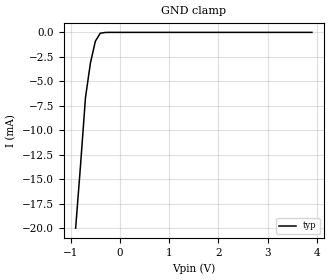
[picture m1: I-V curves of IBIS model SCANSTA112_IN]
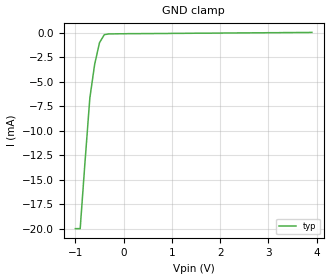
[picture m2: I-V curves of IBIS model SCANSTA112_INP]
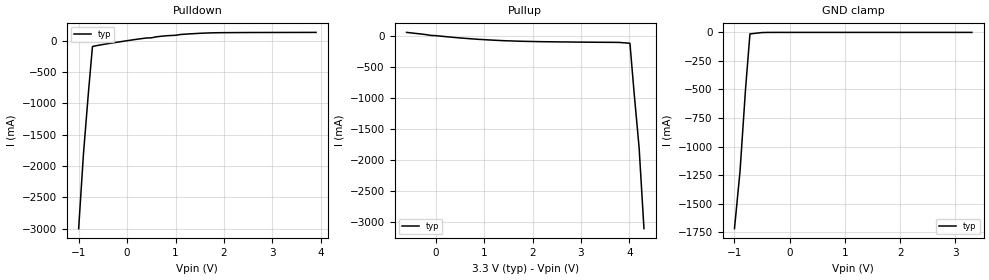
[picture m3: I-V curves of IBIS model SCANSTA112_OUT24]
| Texas Instruments Incorporated
| SCANSTA112 7-Port Multidrop IEEE 1149.1 (JTAG) Multiplexer
| Marketing part#   Voltage Range   Package-type   #pins/pkg drawing
| SCANSTA112VS   3.0V - 3.6V   TQFP   100/NEZ
| SCANSTA112SM   3.0V - 3.6V   NFBGA   100/NZD
[IBIS Ver]   4.1
[File name]   scansta112.ibs
[File Rev]   1.0
[Date]   04/11/13
[Source]   File originated at National Semiconductor Corporation
   System Test Access Group/Enhanced Solutions Division
   All data based on simulations, except where specified.
[Notes]   Revision History
   Rev 1.0: 04/11/2013
   - Model based on SCANSTA101 buffer models. Only nom available.
   Since these models are based on a related device, accuracy is not assured.
[Disclaimer]  This model is designed as an aid for customers of Texas Instruments
 TI and its licensors and suppliers make no warranties, either expressed
 or implied, with respect to this  model, including the warranties of
 merchantability or fitness for a particular purpose.
 The model is provided solely on an "as is" basis. The entire risk as to
 its quality and performance is with the customer.
[Copyright] (C)Copyright 2013 Texas Instruments Incorporated.
   All rights reserved.
| Component SCANSTA112NZD 100 pin NFBGA
[Component]  SCANSTA112NZD
[Manufacturer]  Texas Instruments
[Package]
|   typ   min   max
R_pkg   65.0m   NA   NA
L_pkg   1.50nH   NA   NA
C_pkg   0.08pF   NA   NA
[Pin]   signal_name   model_name   R_pin   L_pin   C_pin
A1   S0   SCANSTA112_IN
A2   TCK06   SCANSTA112_OUT24
A3   TDO06   SCANSTA112_OUT12
A4   VCC   POWER
A5   TMS04   SCANSTA112_OUT24
A6   GND   GND
A7   TCK04   SCANSTA112_OUT24
A8   TMS04   SCANSTA112_OUT24
A9   VCC   POWER
A10   TDO03   SCANSTA112_OUT12
B1   GND   GND
B2   S1   SCANSTA112_IN
B3   GND   GND
B4   TDI06   SCANSTA112_INP
B5   TCK04   SCANSTA112_OUT24
B6   TDO05   SCANSTA112_OUT12
B7   TRST04B   SCANSTA112_OUT24
B8   TCK03   SCANSTA112_OUT24
B9   TMS03   SCANSTA112_OUT24
B10   TRIST02   SCANSTA112_OUT12
C1   S7   SCANSTA112_IN
C2   S3   SCANSTA112_IN
C3   VCC   POWER
C4   TMS06   SCANSTA112_OUT24
C5   TRST05B   SCANSTA112_OUT24
C6   TDO04   SCANSTA112_OUT12
C7   TDI04   SCANSTA112_INP
C8   GND   GND
C9   VCC   POWER
C10   TCK02   SCANSTA112_OUT24
D1   ADDMASK   SCANSTA112_IN
D2   TRANS   SCANSTA112_IN
D3   S5   SCANSTA112_IN
D4   S4   SCANSTA112_IN
D5   TRST06B   SCANSTA112_OUT24
D6   TRST03B   SCANSTA112_OUT24
D7   TRIST03   SCANSTA112_OUT12
D8   TRST02B   SCANSTA112_OUT24
D9   TMS02   SCANSTA112_OUT24
D10   GND   GND
E1   VCC   POWER
E2   LSPsel0   SCANSTA112_IN
E3   S6   SCANSTA112_IN
E4   S2   SCANSTA112_IN
E5   LSPsel1   SCANSTA112_IN
E6   TDI05   SCANSTA112_INP
E7   TDI03   SCANSTA112_INP
E8   TDO02   SCANSTA112_OUT12
E9   TDI02   SCANSTA112_INP
E10   A101   SCANSTA112_IN
F1   OE_B   SCANSTA112_IN
F2   LSPsel2   SCANSTA112_IN
F3   LSPsel3   SCANSTA112_IN
F4   SB/SB   SCANSTA112_IN
F5   A0B1   SCANSTA112_INP
F6   A001   SCANSTA112_IN
F7   RESETB   SCANSTA112_IN
F8   TCK01   SCANSTA112_OUT24
F9   Y001   SCANSTA112_OUT12
F10   VCC   POWER
G1   GND   GND
G2   LSPsel4   SCANSTA112_IN
G3   LSPsel6   SCANSTA112_IN
G4   TRSTB0B   SCANSTA112_IO24
G5   A0B0   SCANSTA112_INP
G6   A1B1   SCANSTA112_INP
G7   TDO01   SCANSTA112_OUT12
G8   TMS01   SCANSTA112_OUT24
G9   Y101   SCANSTA112_OUT12
G10   TRIST01   SCANSTA112_OUT12
H1   LSPsel5   SCANSTA112_IN
H2   VCC   POWER
H3   GND   GND
H4   TMSB0   SCANSTA112_IO24
H5   A1B0   SCANSTA112_INP
H6   TRSTB1B   SCANSTA112_IO24
H7   TRISTB1   SCANSTA112_OUT12
H8   VCC   POWER
H9   TDI01   SCANSTA112_INP
H10   TRST01B   SCANSTA112_OUT24
J1   MPseLB1   SCANSTA112_IN
J2   TDOB0   SCANSTA112_IO12
J3   TCKB0   SCANSTA112_IO24
J4   Y1B0   SCANSTA112_OUT12
J5   TDOB1   SCANSTA112_IO12
J6   TCKB1   SCANSTA112_IO24
J7   TMSB1   SCANSTA112_IO24
J8   GND   GND
J9   TLR_TRST6   SCANSTA112_IN
J10   GND   GND
K1   TDIB0   SCANSTA112_INP
K2   VCC   POWER
K3   TRISTB0   SCANSTA112_OUT12
K4   Y0B0   SCANSTA112_OUT12
K5   GND   GND
K6   TDIB1   SCANSTA112_INP
K7   VCC   POWER
K8   Y1B1   SCANSTA112_OUT12
K9   Y0B1   SCANSTA112_OUT12
K10   TLR_TRST   SCANSTA112_IN
| Component SCANSTA112NEZ 100 pin TQFP
[Component]  SCANSTA112NEZ
[Manufacturer]  Texas Instruments
[Package]
|   typ   min   max
R_pkg   65.0m   NA   NA
L_pkg   1.50nH   NA   NA
C_pkg   0.08pF   NA   NA
[Pin]   signal_name   model_name   R_pin   L_pin   C_pin
1   S0   SCANSTA112_IN
2   S1   SCANSTA112_IN
3   VDD   POWER
4   S2   SCANSTA112_IN
5   S3   SCANSTA112_IN
6   S4   SCANSTA112_IN
7   S5   SCANSTA112_IN
8   GND   GND
9   S6   SCANSTA112_IN
10   S7   SCANSTA112_IN
11   ADDMASK   SCANSTA112_IN
12   TRANS   SCANSTA112_IN
13   VDD   POWER
14   OE_B   SCANSTA112_IN
15   LSPsel0   SCANSTA112_IN
16   LSPsel1   SCANSTA112_IN
17   LSPsel2   SCANSTA112_IN
18   GND   GND
19   LSPsel3   SCANSTA112_IN
20   LSPsel4   SCANSTA112_IN
21   LSPsel5   SCANSTA112_IN
22   LSPsel6   SCANSTA112_IN
23   VDD   POWER
24   MPseLB1   SCANSTA112_IN
25   SB/SB   SCANSTA112_IN
26   TDIB0   SCANSTA112_INP
27   TDOB0   SCANSTA112_IO12
28   GND   GND
29   A0B0   SCANSTA112_INP
30   TCKB0   SCANSTA112_IO24
31   TRSTB0B   SCANSTA112_IO24
32   TMSB0   SCANSTA112_IO24
33   VDD   POWER
34   A1B0   SCANSTA112_INP
35   TRISTB0   SCANSTA112_OUT12
36   Y0B0   SCANSTA112_OUT12
37   Y1B0   SCANSTA112_OUT12
38   GND   GND
39   TDIB1   SCANSTA112_INP
40   TDOB1   SCANSTA112_IO12
41   A0B1   SCANSTA112_INP
42   TCKB1   SCANSTA112_IO24
43   VCC   POWER
44   TRSTB1B   SCANSTA112_IO24
45   TMSB1   SCANSTA112_IO24
46   Y1B1   SCANSTA112_OUT12
47   TRISTB1   SCANSTA112_OUT12
48   GND   GND
49   Y0B1   SCANSTA112_OUT12
50   A1B1   SCANSTA112_INP
51   TLR_TRST   SCANSTA112_IN
52   TLR_TRST6   SCANSTA112_IN
53   VCC   POWER
54   RESETB   SCANSTA112_IN
55   TDI01   SCANSTA112_INP
56   TDO01   SCANSTA112_OUT12
57   TMS01   SCANSTA112_OUT24
58   GND   GND
59   TCK01   SCANSTA112_OUT24
60   TRST01B   SCANSTA112_OUT24
61   TRIST01   SCANSTA112_OUT12
62   Y101   SCANSTA112_OUT12
63   VCC   POWER
64   A101   SCANSTA112_IN
65   Y001   SCANSTA112_OUT12
66   A001   SCANSTA112_IN
67   TDI02   SCANSTA112_INP
68   GND   GND
69   TDO02   SCANSTA112_OUT12
70   TMS02   SCANSTA112_OUT24
71   TCK02   SCANSTA112_OUT24
72   TRST02B   SCANSTA112_OUT24
73   VCC   POWER
74   TRIST02   SCANSTA112_OUT12
75   TDI03   SCANSTA112_INP
76   TDO03   SCANSTA112_OUT12
77   TMS03   SCANSTA112_OUT24
78   GND   GND
79   TRST03B   SCANSTA112_OUT24
80   TCK03   SCANSTA112_OUT24
81   TRIST03   SCANSTA112_OUT12
82   TDI04   SCANSTA112_INP
83   VCC   POWER
84   TDO04   SCANSTA112_OUT12
85   TMS04   SCANSTA112_OUT24
86   TCK04   SCANSTA112_OUT24
87   TRST04B   SCANSTA112_OUT24
88   GND   GND
89   TMS05   SCANSTA112_OUT24
90   TDO05   SCANSTA112_OUT12
91   TDI05   SCANSTA112_INP
92   TCK05   SCANSTA112_OUT24
93   VCC   POWER
94   TRST05B   SCANSTA112_OUT24
95   TDI06   SCANSTA112_INP
96   TDO06   SCANSTA112_OUT12
97   TMS06   SCANSTA112_OUT24
98   GND   GND
99   TCK06   SCANSTA112_OUT24
100   TRST06B   SCANSTA112_OUT24
| Models and submodels in the file (6): SCANSTA112_IN (Input), SCANSTA112_INP (Input), SCANSTA112_OUT24 (3-state), SCANSTA112_IO24 (I/O), SCANSTA112_OUT12 (3-state), SCANSTA112_IO12 (I/O)
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|   Input MODEL
[Model]   SCANSTA112_IN
Model_type   Input
Vinh = 2.0
Vinl = 0.8
|   typ   min   max
C_comp   5.00pF   NA   NA
|   typ   min   max
[Temperature Range]   25.0   NA   NA
[Voltage range]   3.3V   NA   NA
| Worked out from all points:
|   GND clamp passes 1 mA (typ) near -0.50 V on its own axis
[GND_clamp]
| Voltage   I(typ)   I(min)   I(max)
-900mV    -19.99mA   NA         NA
-800mV    -13.52mA   NA         NA
-700mV    -6.65mA    NA         NA
-600mV    -3.14mA    NA         NA
-500mV    -910uA     NA         NA
-400mV    -90uA      NA         NA
-200mV    0A         NA         NA
3.9V      0A         NA         NA
[Power_clamp]
| Voltage   I(typ)   I(min)   I(max)
-3.3V     0A         NA         NA
3.3V      0A         NA         NA
|   Input Pull-up MODEL
[Model]   SCANSTA112_INP
Model_type   Input
Vinh = 2.0
Vinl = 0.8
|   typ   min   max
C_comp   5.00pF   NA   NA
|   typ   min   max
[Temperature Range]   25.0   NA   NA
[Voltage range]   3.3V   NA   NA
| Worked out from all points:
|   GND clamp passes 1 mA (typ) near -0.50 V on its own axis
[GND_clamp]
| Voltage   I(typ)   I(min)   I(max)
-1V       -19.99mA   NA         NA
-900mV    -19.99mA   NA         NA
-800mV    -13.18mA   NA         NA
-700mV    -6.68mA    NA         NA
-600mV    -3.23mA    NA         NA
-500mV    -1.03mA    NA         NA
-400mV    -210uA     NA         NA
-300mV    -130uA     NA         NA
3.9V      20uA       NA         NA
[Power_clamp]
| Voltage   I(typ)   I(min)   I(max)
-3.3V     0A         NA         NA
3.3V      0A         NA         NA
|   3-State Output 24mA MODEL
[Model]   SCANSTA112_OUT24
Model_type   3-state
Vmeas =   1.25
| Variable   typ   min   max
C_comp   5.00pF   NA   NA
|   typ   min   max
[Temperature Range]   25.0   NA   NA
[Voltage range]   3.3V   NA   NA
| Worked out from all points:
|   slope of the pulldown table from 0 to 0.495 V, typ, clamps not added: 10.9 ohm
|   slope of the pullup table from 0 to 0.495 V, typ, clamps not added: 13.5 ohm
|   GND clamp passes 1 mA (typ) near -0.46 V on its own axis
[Pulldown]
| Voltage   I(typ)   I(min)   I(max)
-1V       -3A        NA         NA
-900mV    -1.8A      NA         NA
-800mV    -844mA     NA         NA
-715mV    -93.6mA    NA         NA
300mV     33mA       NA         NA
1.3V      109.2mA    NA         NA
1.9V      127.5mA    NA         NA
3.9V      132.3mA    NA         NA
[Pullup]
| Voltage   I(typ)   I(min)   I(max)
-600mV    52mA       NA         NA
500mV     -37mA      NA         NA
1.4V      -81mA      NA         NA
3.765V    -108.6mA   NA         NA
4.01V     -122mA     NA         NA
4.1V      -947mA     NA         NA
4.2V      -1.8A      NA         NA
4.3V      -3.1A      NA         NA
[GND_clamp]
| Outputs in Tri-state.
| Voltage   I(typ)   I(min)   I(max)
-1V       -1.72A     NA         NA
-900mV    -1.22A     NA         NA
-800mV    -498mA     NA         NA
-720mV    -13mA      NA         NA
-400mV    -240uA     NA         NA
3.3V      586pA      NA         NA
[POWER_clamp]
| Voltage   I(typ)   I(min)   I(max)
-3.3V     0A         NA         NA
3.3V      0A         NA         NA
[Ramp]
|   typ   min   max
dV/dt_r   1.889/1.12n   NA   NA
dV/dt_f   1.889/0.69n   NA   NA
|[Cload]   30p
R_load = 500ohms
